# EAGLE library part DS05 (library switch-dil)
DIL/CODE SWITCH
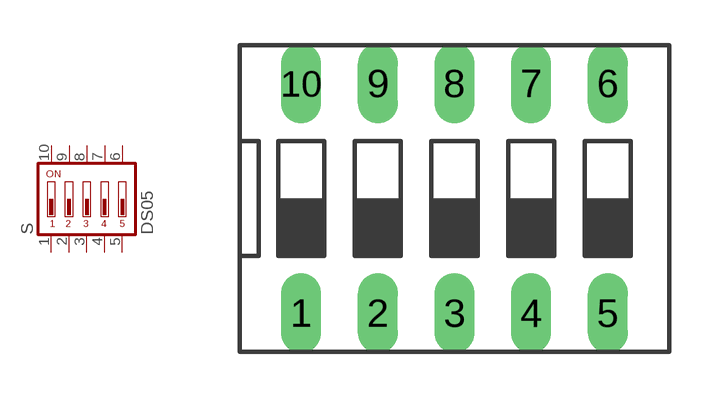
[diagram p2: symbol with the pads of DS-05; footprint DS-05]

Designator prefix S

## DS05 (OC_FARNELL: 1255225; OC_NEWARK: unknown)  [DS-05]
1  1  pas
2  2  pas
3  3  pas
4  4  pas
5  5  pas
6  6  pas
7  7  pas
8  8  pas
9  9  pas
10  10  pas

## Footprint DS-05 (pad centres in mm)
DIL/CODE SWITCH Mors distributor Buerklin, 17G556
drill 0.813 long: 1 -5.08,-3.81; 2 -2.54,-3.81; 3 0,-3.81; 4 2.54,-3.81; 5 5.08,-3.81; 6 5.08,3.81; 7 2.54,3.81; 8 0,3.81; 9 -2.54,3.81; 10 -5.08,3.81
